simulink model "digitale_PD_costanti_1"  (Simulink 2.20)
settings: Solver=VariableStepDiscrete  StartTime=0.0  StopTime=10.0  RelTol=1e-3  AbsTol=1e-6
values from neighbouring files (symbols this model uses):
  Kalfa = DT/Ti    [pidin.m]
  Kbeta = N*Kgamma    [pidin.m]
undefined symbols (not defined in the file or in its folder): Kp, T

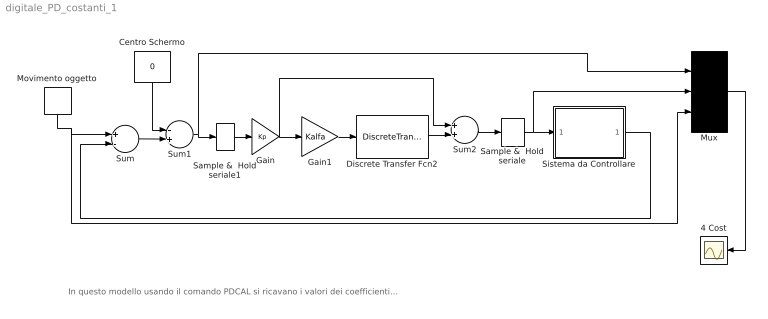
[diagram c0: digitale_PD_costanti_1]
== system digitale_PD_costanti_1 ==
  note: In questo modello usando il comando PDCAL si ricavano i valori dei coefficienti Kbeta Kalfa dalla precedente definizione dei parametri T Td Kp N........ vedi file digitale_PD_costanti
  4 Cost : Scope
  Centro Schermo : Constant  Orientation=down  Value=0
  Discrete Transfer Fcn2 : DiscreteTransferFcn  Numerator=[1 -1]  Denominator=[1 Kbeta]  SampleTime=.005
  Gain : Gain  Gain=Kp
  Gain1 : Gain  Gain=Kalfa
  Movimento oggetto : DiscretePulseGenerator  Orientation=down  Amplitude=47.5  Period=100  PulseWidth=100  PhaseDelay=10  SampleTime=.1
  Mux : Mux  Inputs=3
  Sample &  Hold seriale : ZeroOrderHold  SampleTime=.260
  Sample &  Hold seriale1 : ZeroOrderHold  SampleTime=T
  Sistema da Controllare : Subsystem
  Sum : Sum  Inputs=+-
  Sum1 : Sum  Inputs=-+
  Sum2 : Sum  Inputs=++
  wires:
  Sum/1 -> Sum1/2
  Centro Schermo/1 -> Sum1/1
  Sum1/1 -> Mux/1, Sample &  Hold seriale1/1
  Gain1/1 -> Discrete Transfer Fcn2/1
  Sistema da Controllare/1(Out1) -> Sum/2
  Discrete Transfer Fcn2/1 -> Sum2/2
  Sum2/1 -> Sample &  Hold seriale/1
  Sample &  Hold seriale/1 -> Sistema da Controllare/1(In1), Mux/2
  Movimento oggetto/1 -> Sum/1, Mux/3
  Mux/1 -> 4 Cost/1
  Gain/1 -> Gain1/1, Sum2/1
  Sample &  Hold seriale1/1 -> Gain/1

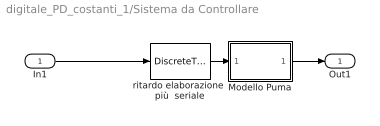
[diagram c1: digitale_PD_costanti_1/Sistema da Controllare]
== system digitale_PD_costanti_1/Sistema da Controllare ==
  In1 : Inport  Port=1  PortWidth=-1  SampleTime=-1
  Modello Puma : Subsystem  Description=Modello Puma
  ritardo elaborazione  più  seriale : DiscreteTransferFcn  Numerator=1  Denominator=[1 0 0 0 0]  SampleTime=.032
  Out1 : Outport  Port=1
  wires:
  ritardo elaborazione  più  seriale/1 -> Modello Puma/1(In1)
  Modello Puma/1(Out1) -> Out1/1
  In1/1 -> ritardo elaborazione  più  seriale/1

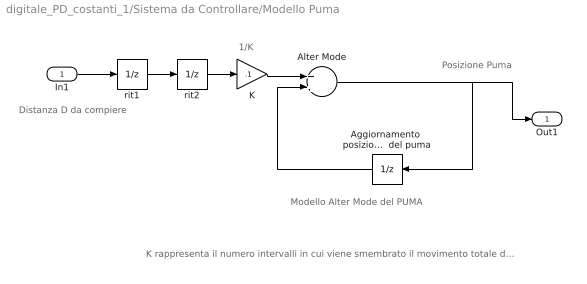
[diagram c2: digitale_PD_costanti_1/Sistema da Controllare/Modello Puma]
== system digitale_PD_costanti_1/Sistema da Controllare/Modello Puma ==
  note: Posizione Puma
  note: Modello Alter Mode del PUMA
  note: 1/K
  note: K rappresenta il numero intervalli in cui viene smembrato il movimento totale da compiere, dopo K time-slice (del PUMA) si ottiene che si e' compiuto proprio la distanza D trasmessa.
  note: Distanza D da compiere
  In1 : Inport  Port=1  PortWidth=-1  SampleTime=-1
  Aggiornamento  posizione   Il sample-time di questo blocco rappresenta la TIME-SLICE  del puma : UnitDelay  Orientation=left  X0=0  SampleTime=.032
  Alter Mode : Sum  Inputs=++
  K : Gain  Gain=.1
  rit1 : UnitDelay  X0=0  SampleTime=.032
  rit2 : UnitDelay  X0=0  SampleTime=.032
  Out1 : Outport  Port=1
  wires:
  K/1 -> Alter Mode/1
  Aggiornamento  posizione   Il sample-time di questo blocco rappresenta la TIME-SLICE  del puma/1 -> Alter Mode/2
  Alter Mode/1 -> Out1/1, Aggiornamento  posizione   Il sample-time di questo blocco rappresenta la TIME-SLICE  del puma/1
  In1/1 -> rit1/1
  rit1/1 -> rit2/1
  rit2/1 -> K/1
